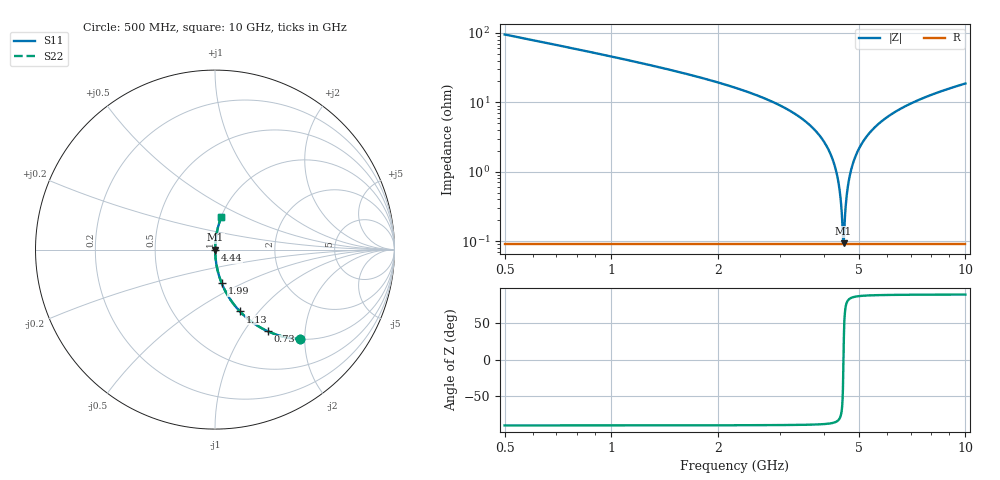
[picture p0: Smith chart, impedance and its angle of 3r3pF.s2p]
! Created Fri Jan 10 15:52:38 2014
# hz S db R 50
! 2 Port Network Data from SP1.SP block
! freq  dbS11  angS11  dbS21  angS21  dbS12  angS12  dbS22  angS22
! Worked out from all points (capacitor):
!   951 points, 500 MHz to 10 GHz, reference 50 ohm
!   read as one part in series: C = 3.3 pF near 540 MHz
!   lowest |Z| = 92.3 mohm at 4.53 GHz (marker M1)
!   series resonance near 4.527 GHz, so ESL is about 370 pH
!   S11 on the Smith chart (normalised r, x): 500 MHz: 1.00, -1.91; 730 MHz: 1.00, -1.29; 1.13 GHz: 1.00, -0.80; 1.99 GHz: 1.00, -0.39; 4.44 GHz: 1.00, -0.01; 10 GHz: 1.00, +0.37
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5e8  -3.23 -46.4  -2.81 43.6  -2.81 43.6  -3.23 -46.4
7.3e8  -5.34 -57.2  -1.51 32.7  -1.51 32.7  -5.34 -57.2
1.13e9  -8.61 -68.1  -0.65 21.8  -0.65 21.8  -8.61 -68.1
1.99e9  -14.35 -78.7  -0.17 11.1  -0.17 11.1  -14.35 -78.7
2.09e9  -14.97 -79.4  -0.15 10.3  -0.15 10.3  -14.97 -79.4
3.07e9  -21.47 -84.5  -0.04 4.8  -0.04 4.8  -21.47 -84.5
3.67e9  -26.94 -86.3  -0.02 2.6  -0.02 2.6  -26.94 -86.3
3.97e9  -31.05 -86.5  -0.01 1.6  -0.01 1.6  -31.05 -86.5
4.19e9  -35.65 -85.9  -0.01 0.9  -0.01 0.9  -35.65 -85.9
4.34e9  -40.90 -83.7  -0.01 0.5  -0.01 0.5  -40.90 -83.7
4.44e9  -47.50 -77.3  -0.01 0.2  -0.01 0.2  -47.50 -77.3
4.5e9  -56.18 -54.1  -0.01 0.1  -0.01 0.1  -56.18 -54.1
4.53e9  -60.70 9.7  -0.01 -0.0  -0.01 -0.0  -60.70 9.7
4.55e9  -56.94 50.2  -0.01 -0.1  -0.01 -0.1  -56.94 50.2
4.64e9  -45.45 79.9  -0.01 -0.3  -0.01 -0.3  -45.45 79.9
4.75e9  -39.75 84.3  -0.01 -0.6  -0.01 -0.6  -39.75 84.3
4.95e9  -34.39 86.2  -0.01 -1.1  -0.01 -1.1  -34.39 86.2
5.25e9  -29.99 86.5  -0.01 -1.8  -0.01 -1.8  -29.99 86.5
5.89e9  -24.94 85.8  -0.02 -3.2  -0.02 -3.2  -24.94 85.8
6.84e9  -20.91 84.3  -0.04 -5.2  -0.04 -5.2  -20.91 84.3
8.42e9  -17.11 81.6  -0.09 -8.0  -0.09 -8.0  -17.11 81.6
1e10  -14.71 79.1  -0.16 -10.6  -0.16 -10.6  -14.71 79.1
